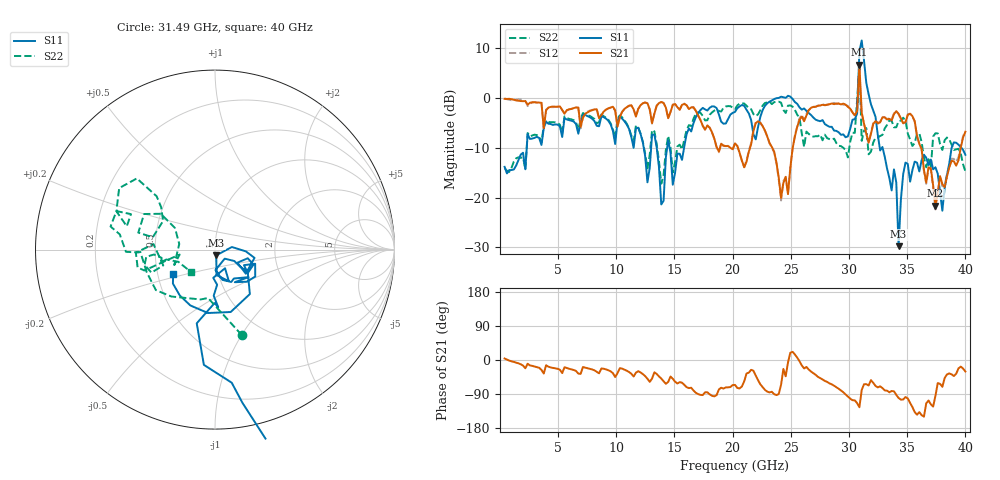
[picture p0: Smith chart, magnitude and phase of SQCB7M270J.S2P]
! Network Analyzer HP8722ES.07.66: Jul 25, 2000 Serial No. US39175408
! 27 Oct 2004  08:55:51
! Frequency  S11  S21  S12  S22
# HZ  S  DB R  50
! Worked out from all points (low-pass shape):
!   201 points, 400 MHz to 40 GHz, reference 50 ohm
!   highest |S21| = 6.67 dB at 30.89 GHz (marker M1); lowest = -21.6 dB at 37.43 GHz (marker M2)
!   |S21| within 3 dB of the highest: 30.82833 GHz to 30.95374 GHz (125.4 MHz wide, 0.406 % of centre)
!   lowest |S11| = -29.7 dB at 34.26 GHz (marker M3), VSWR 1.07, Z = 50.6 - j3.22 ohm
!   |S11| at or under -10 dB: start of sweep to 2.303 GHz; 14.58 GHz to 15.82 GHz (1.243 GHz wide, 8.18 % of centre); 32.89 GHz to 38.82 GHz (5.93 GHz wide, 16.5 % of centre)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
!   |S22| runs from -17.2 to 6.6 dB; largest |S21 - S12| = 0.61
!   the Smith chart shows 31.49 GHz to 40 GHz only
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4e8  -13.82 -90.7  -0.17 4.0  -0.07 5.3  -14.08 -85.7
7.132e9  -3.30 -109.5  -3.92 -18.4  -4.00 -19.7  -3.01 -98.7
1.3666e10  -13.88 -125.7  -1.02 -43.3  -0.96 -43.7  -12.69 -93.0
2.02e10  -2.80 -6.8  -9.11 -65.6  -9.06 -66.1  -2.26 -9.3
2.1982e10  -8.30 0.5  -5.04 -41.2  -4.86 -42.8  -3.63 -14.2
2.3566e10  -0.22 1.7  -10.77 -90.1  -10.97 -90.9  -0.83 -29.0
2.416e10  0.26 -7.6  -20.08 -65.3  -20.57 -63.1  -0.94 -51.2
2.515e10  -0.19 -13.6  -10.12 21.6  -10.25 17.8  -1.74 -92.6
2.6932e10  -3.93 -21.4  -1.78 -34.9  -1.81 -36.1  -7.76 142.0
2.9902e10  -7.71 11.1  -1.78 -96.4  -1.60 -97.3  -11.93 105.6
3.0694e10  -3.15 9.4  -2.66 -113.8  -2.57 -113.5  -0.41 124.1
3.0892e10  9.40 -17.6  6.67 -124.7  4.02 -131.6  6.60 138.3
3.109e10  11.55 -28.5  -2.95 -79.1  -3.09 -79.8  -8.61 -106.3
3.1288e10  7.51 -49.5  -5.15 -64.0  -5.21 -64.6  -6.56 -70.5
3.1684e10  0.75 -75.0  -8.97 -67.2  -8.85 -68.6  -11.30 -98.2
3.3466e10  -16.06 -93.6  -4.17 -85.2  -4.09 -87.0  -4.50 167.5
3.406e10  -16.95 -86.6  -2.64 -92.0  -2.61 -93.0  -5.88 165.2
3.4258e10  -29.74 -77.2  -3.18 -100.3  -3.26 -100.7  -4.64 159.0
3.4852e10  -12.96 -11.8  -4.85 -97.6  -4.90 -97.8  -4.60 137.7
3.7426e10  -13.90 -63.4  -21.62 -94.6  -22.38 -91.5  -7.08 -167.0
3.802e10  -22.62 -43.0  -17.26 -70.7  -17.72 -67.5  -10.42 -163.1
4e10  -11.41 -150.0  -6.77 -30.3  -6.69 -32.7  -14.74 -138.1
